(* Logix 5000 Rung export; software revision 16.04 *)

TYPE AFCEModbusGatewayCommand :   // Modbus Gateway Command
STRUCT
   Config : AFCEModbusGatewayConfig;   // Config data to be entered by the user.
   Trigger : BOOL;   // Trigger the Command, when cleared module has responded.
   Data : INT[200];   // Contains modbus data written to the module (write commands)
END_STRUCT
END_TYPE

TYPE AFCEModbusMasterDataType :   // Modbus master data type
STRUCT
   Bit : BOOL;   // bit type
   Word : BOOL;   // word type (16-bit)
   Long : BOOL;   // long integer (32-bit)
   LongRemote : BOOL;   // long integer (32-bit)
END_STRUCT
END_TYPE

TYPE AFCEFlag :   // Flags contains status information updated by ladder and also trigger bits for clock update
STRUCT
   AFCStopped : BOOL;   // Indicates that the module has sent a new input block to be processed by ladder - UPDATED BY LADDER
   AFCInputSequenceNum : INT;   // Meter number (0 -15) associated to blocks 1-16. Used to update "Profile" (meter type and product group.) UPDATED BY LADDER
END_STRUCT
END_TYPE

TYPE AFCEModbusGateway :   // Modbus Gateway
STRUCT
   Command : AFCEModbusGatewayCommand[10];   // Modbus gateway commands - contains setup and modbus data
END_STRUCT
END_TYPE

TYPE AFCEFirmwareVersion :
STRUCT
   Major : SINT;   // Major Version number
   Minor : SINT;   // Minor Version number
   Revision : INT;   // Revision
END_STRUCT
END_TYPE

TYPE AFCEProveConfigEnable :   // Prove controls at enable
STRUCT
   MeterNumber : INT;   // Meter number requested (1-16)
   AutoAcceptProve : BOOL;   // Auto-accept the prove
   AutoContinueProve : BOOL;   // Auto-continue the prove
END_STRUCT
END_TYPE

TYPE AFCEModbusMasterSwap :   // Modbus master swap words/ swap bytes
STRUCT
   SwapWords : BOOL;   // Swap words
   SwapBytes : BOOL;   // Swap bytes
END_STRUCT
END_TYPE

TYPE AFCEUtil :   // Used for internal ladder logic usage. These values must not be changed by user application.
STRUCT
   Flags : AFCEFlag;   // Wallclock update commands
   CycleCounter : INT;   // Reflects current block ID calculated by ladder to be sent to the module
   Buffer : AFCEUtilBuffer;
   Block : AFCEUtilBlock;
END_STRUCT
END_TYPE

TYPE AFCENetworkUTIL :
STRUCT
   State : INT;
   Buffer : SINT[240];
   TimeoutTimer : TIMER;
   TimeoutState : INT;
END_STRUCT
END_TYPE

TYPE AFCEProveConfigAccept :   // Prove controls at accept. If auto-accept is selected must be available at enable
STRUCT
   RequestedInterpolationPoint : INT;   // Requested interpolation point (0 nearest)
   ApplyMFChangeAllStreams : BOOL;   // Apply change in meter factor to all streams
   ApplyMFChangeCurve : BOOL;   // Apply change in meter factor to all curve points
   ApplyNewMF : BOOL;   // CApply new meter factor
END_STRUCT
END_TYPE

TYPE AFCEUtilBlockNonInterrupt :
STRUCT
   Now : BOOL;
   ModbusMasterCommand : BOOL;
   ModbusMasterResponse : BOOL;
   Archive : DINT;
   Prover : BOOL;
   PassThru : BOOL;
   Calibration : BOOL;
END_STRUCT
END_TYPE

TYPE AFCEProve :   // Prove
STRUCT
   Process : AFCEProveProcess;   // Process Variables
   Signals : AFCEProveSignals;   // AFC Prove Signals (triggers the proving update)
   Config : AFCEProveConfig;   // AFC Prove Control (configuration settings)
   PulseCounts : AFCEProvePulseCount;   // Pulse counts to be updated at the end of the run/pass
   ConfigInput : AFCEProveInputConfig;   // AFC prover input configuration
   Status : AFCEProveStatus;   // AFC prover status
   ErrorCode : INT;   // Prove error code
   ProveControlsEcho : INT;   // AFC module Echos the state of the Prove Controls
   RequestedMeterEcho : INT;   // AFC module Echos the Meter number requested
   RequestedCurvePointEcho : INT;   // AFC module Echos the requested Curve Point
   RunResults : AFCEProveRunResults;   // Prove and run results
   ProveEnabled : BOOL;   // ON if prove is enabled. This flag is coped from inputbuffer[247]
END_STRUCT
END_TYPE

TYPE AFCEWallclock :
STRUCT
   GetAFCTime : BOOL;   // Get current AFC Time
   SetAFCTimeFromPLCTime : BOOL;   // Set AFC time from PLC time. Updates current AFC time
   EnableLocalDateTime : BOOL;   // Enable Local Date Time.
   AFCTime : AFCETime;   // Coordinated Universal Time. Updated by either getting or setting AFC time.
END_STRUCT
END_TYPE

TYPE AFCESiteStatus :   // Site status bits - contains general information about the module - not meter specific
STRUCT
   AFCActive : BOOL;   // AFC active
   ChecksumAlarms : BOOL;   // Checkum alarm active
   Reserved2 : BOOL;
   Reserved3 : BOOL;
   PLCHalted : BOOL;   // PLC in program mode or missing
   CfgChanged : BOOL;   // Configuration changed
   Powerup : BOOL;   // Module powered up
   ColdStart : BOOL;   // Module performed cold start (BBRAM initialized)
   ModbusMasterPending : BOOL;   // Modbus Master Poll Pending
   ModbusMasterComplete : BOOL;   // Modbus Master Poll Complete
   ModbusPassThruPending : BOOL;   // Modbus Pass-thru Input Pending
   CalibrationRequest : BOOL;   // Calibration request from module
   ProverEnabled : BOOL;   // Prover Enabled
   Reserved13 : BOOL;
   Reserved14 : BOOL;
   Reserved15 : BOOL;
END_STRUCT
END_TYPE

TYPE AFCEModbusMasterConfig :   // Modbus master command settings
STRUCT
   Enable : BOOL;   // Set to 1 to enable command (0=disable)
   FunctionType : BOOL;   // Set to 1 to select write command (0=read command)
   RegisterBank : BOOL;   // Set to 1 to select input register (0=holding register)
   DataType : AFCEModbusMasterDataType;   // Select data type format
   SwapOption : AFCEModbusMasterSwap;   // Select byte and word swap (1 = swap, 0 = no swap)
   TypeSwap : INT;   // This value is calculated by ladder logic and must not be modified by user
   SlaveAddress : INT;   // Modbus slave address of remote device
   ModbusAddress : INT;   // Modbus data address on remote slave
   ElementCount : INT;   // Number of data elements (125 words)
   TransactionID : INT;   // Transaction ID. This value is returned to the ReturnedTransaction ID when the response has been received.
END_STRUCT
END_TYPE

TYPE AFCEProvePulseCount :   // Values to be supplied at the end of the pass/run
STRUCT
   Meter : DINT;   // Meter pulse count
   MasterMeter : DINT;   // Master meter pulse count
END_STRUCT
END_TYPE

TYPE AFCEUtilBuffer :   // Buffer
STRUCT
   Input : INT[250];   // Input buffer contains the complete block to be copied from the module
   Output : INT[248];   // Output buffer contains data the complete block to be copied to the module
   Process : INT[240];
   ArchiveDay : INT[98];
   ArchiveHour : INT[98];
   Prove : INT[26];
   Analysis : INT[198];
   MeterEnableDisable : INT[4];
   StreamEnable : INT[48];
   StreamDisable : INT[48];
   StreamSelect : INT[32];
   MeterSignals : INT[32];
   Calibration : INT[36];
END_STRUCT
END_TYPE

TYPE AFCEModbusPassThru :   // AFC Modbus Pass-thru
STRUCT
   Enable : BOOL;   // Set to 1 to enable pass-thru functionality (requires AFC Manager setting)
   MessagePresent : BOOL;   // Message present in the response block
   GetMessage : BOOL;   // Get the pass-thru message. When the bit is cleared the message has been transferred to the PLC.
   FunctionBitWrite : BOOL;   // Function bit write
   OverflowError : BOOL;   // Overflow error flag
   ModbusAddress : INT;   // Destination modbus address
   RegisterCount : INT;   // Number of elements associated to command
   ReadDataWord : INT[125];   // Contains received data for word commands
   ReadDataBit : AFCEModbusPassThruBitData;   // Contains received data for bit commands
END_STRUCT
END_TYPE

TYPE AFCEModbusGatewayConfig :   // Modbus Ggateway Configuration
STRUCT
   Enable : BOOL;   // Set to 1 to enable modbus gateway command (0=disable)
   StartRegister : DINT;   // Start modbus address
   RegisterCount : INT;   // Word count (200 max)
   FunctionType : BOOL;   // 0 = read command, 1 = write command
   RegisterType : BOOL;   // 0 = holding register, 1 = input register
   SlaveType : BOOL;   // 0 = primary slave, 1 = virtual slave
END_STRUCT
END_TYPE

TYPE AFCEUtilBlockInterrupt :
STRUCT
   Now : BOOL;
   ModbusGateway : DINT;
   EnableDisable : BOOL;
   Analysis : DINT;
END_STRUCT
END_TYPE

TYPE AFCEModbusMasterCommand :   // Modbus Master Command
STRUCT
   Config : AFCEModbusMasterConfig;   // Modbus Master Configuration
   ErrorCode : INT;   // Error Code associated to Modbus Master Command
   Pending : BOOL;   // Pending Modbus Master Command - waiting for Modbus Response
   ReturnedTransactionID : DINT;   // Changes to Config.TransactionID value when response has returned.
   Data : INT[100];   // Read or Write Data
END_STRUCT
END_TYPE

TYPE AFCEProveStatus :   // Status of the prove (returned from the module to the processor)
STRUCT
   ProveAccepted : BOOL;   // Prove was accepted
   MeterFactorApplied : BOOL;   // Meter factor was applied
   MFAppliedToCurve : BOOL;   // Meter factor was applied to all points in the curve
   MFAppliedToStreams : BOOL;   // Meter factor was applied to all streams
   ProveRejectedByCommand : BOOL;   // Prove was rejected by command
   ProveRejectedNoRuns : BOOL;   // Prove was rejected - empty prove (no runs)
   ProveRejectedDivideBy0 : BOOL;   // Prove was rejected - divide by 0
   ProveEnabled : BOOL;   // Prove is enabled
   ProvingRunInProgress : BOOL;   // Proving run is in progress
   ProveRejectedAbort : BOOL;   // Prove rejected: abort
   ProvePaused : BOOL;   // Prove is paused
   RunCancelled : BOOL;   // Run Is cancelled
   RunTimedOut : BOOL;   // Run timed out
END_STRUCT
END_TYPE

TYPE AFCETime :   // AFC time format used for wallclock update.
STRUCT
   Year : DINT;   // Year
   Month : DINT;   // Month
   Day : DINT;   // Day
   Hour : DINT;   // Hour
   Minute : DINT;   // Minute
   second : DINT;   // Seconds
END_STRUCT
END_TYPE

TYPE AFCEModbusPassThruBitData :   // AFC Modbus Pass-thru Bit Data
STRUCT
   Data : BOOL[2016];   // Contains received data for bit commands
END_STRUCT
END_TYPE

TYPE AFCENetworkConfig :
STRUCT
   GatewayIndex : DINT;
   Physical_Interface_IP : INT[4];
   Physical_Interface_Network_Prefix : SINT;
   Default_Gateway_IP : INT[4];   // The IP address of the gateway. Must be in the same network as the web interface, or null.
   Server1_Network_Prefix : SINT;   // The network prefix length (number of subnet mask bits) of the interface for server 1; a number between 0 and 32.
   Server1_MBAP_Port : DINT;   // The Modbus-TCP port for server 1; 502, or a number between 1024 and 65535.
   Server1_Listener_IP : INT[4];   // The IP address of the network interface for server 1.
END_STRUCT
END_TYPE

TYPE AFCEProveSequencing :   // AFC prove sequencing tag for phase selection and ball positioning
STRUCT
   Phase : AFCEProvePhaseBitmap;   // AFC phase sequencing
   BallPositionReady : BOOL;   // Ball position: Ready (Udir & Bdir only; fwd leg Bdir)
   BallPositionSealed : BOOL;   // Ball position: Sealed (Udir & Bdir only; fwd leg Bdir)
   BallPositionReadyBwdLeg : BOOL;   // Ball position: Ready bwd leg (Bdir only)
   BallPositionSealedBwdLeg : BOOL;   // Ball position: Sealed bwd leg (Bdir only)
END_STRUCT
END_TYPE

TYPE AFCEModbusMaster :   // Modbus Master. Port 3 must be configured as modbus master through AFC Manager to use this feature.
STRUCT
   Enable : BOOL;   // Enable the modbus master funcionality
   CommandIndex : INT;   // Selects which command index will be executed
   Command : AFCEModbusMasterCommand[10];   // Each command contains a specific modbus request to be sent out of the port
END_STRUCT
END_TYPE

TYPE AFCESiteAlarms :   // Indicates if a meter has any alarms
STRUCT
   Meter1 : BOOL;   // Meter in alarm
   Meter2 : BOOL;   // Meter in alarm
   Meter3 : BOOL;   // Meter in alarm
   Meter4 : BOOL;   // Meter in alarm
   Meter5 : BOOL;   // Meter in alarm
   Meter6 : BOOL;   // Meter in alarm
   Meter7 : BOOL;   // Meter in alarm
   Meter8 : BOOL;   // Meter in alarm
   Meter9 : BOOL;   // Meter in alarm
   Meter10 : BOOL;   // Meter in alarm
   Meter11 : BOOL;   // Meter in alarm
   Meter12 : BOOL;   // Meter in alarm
   Meter13 : BOOL;   // Meter in alarm
   Meter14 : BOOL;   // Meter in alarm
   Meter15 : BOOL;   // Meter in alarm
   Meter16 : BOOL;   // Meter in alarm
END_STRUCT
END_TYPE

TYPE AFCEProveSignals :   // Contains the proving signals that will trigger specific tasks from the module
STRUCT
   EnableProve : BOOL;   // Enables the prove
   AcceptProve : BOOL;   // Accepts the prove
   RejectProve : BOOL;   // Reject the prove
   RunStart : BOOL;   // Starts the run
   RunComplete : BOOL;   // Flags that the run is complete
   RunCancel : BOOL;   // Cancels the run
   RunDelete : BOOL;   // Deletes the run
   PassComplete : BOOL;   // Flag that the pass is complete
   PauseProve : BOOL;   // Pauses the Proving Process
   AbortProve : BOOL;   // Aborts the prove
END_STRUCT
END_TYPE

TYPE AFCEProvePhaseBitmap :   // AFC prove phase bitmap
STRUCT
   NotSelected : BOOL;   // Not selected
   Active : BOOL;   // Active, not counting
   CountingPast1stSwitch : BOOL;   // Counting past 1st switch for Udir and forward leg for Bdir)
   Past2ndSwitchFwdLeg : BOOL;   // Past 2nd switch forward leg (bidirectional only)
   Past1stSwithRetLeg : BOOL;   // Past 1st switch return leg (bidirectional only)
   RunComplete : BOOL;   // Run complete. past 2nd switch.
END_STRUCT
END_TYPE

TYPE AFCEUtilBlock :
STRUCT
   ProcessInput : INT;
   InterruptPending : AFCEUtilBlockInterrupt;
   InterruptComplete : AFCEUtilBlockInterrupt;
   NonInterruptPending : AFCEUtilBlockNonInterrupt;
   NonInterruptComplete : AFCEUtilBlockNonInterrupt;
END_STRUCT
END_TYPE

TYPE AFCEProveProcess :   // Prove process output from processor to the module
STRUCT
   Sequencing : AFCEProveSequencing;   // Prover sequencing
   Temperature : REAL;   // Temperature for Single Probe provers. And Inlet Temperature for Dual Probe Provers.
   OutletTemperature : REAL;   // Outlet Temperature for Provers with Dual Probes.
   SwitchBarTemperature : REAL;   // Switch bar temperature
   Pressure : REAL;   // Pressure for Single Probe provers. And Inlet Pressure for Dual Probe Provers.
   OutletPressure : REAL;   // Outlet Pressure for Provers with Dual Probes.
   ProverDensity : REAL;   // Prover density
END_STRUCT
END_TYPE

TYPE AFCENetwork :
STRUCT
   Read : BOOL;   // Trigger to read network parameters
   Write : BOOL;   // Trigger to write network parameters
   Config : AFCENetworkConfig;   // Network parameters
   Error : INT;   // 0 = OK, -1 = Timeout, -2 = Gateway Index Out of Range
   Util : AFCENetworkUTIL;   // Internal variables
END_STRUCT
END_TYPE

TYPE AFCEProveInputConfig :   // Prove input block results - prover configuration
STRUCT
   Type : INT;   // Prover type
   Options : INT;   // Prover options
   RunsPerProveTotal : INT;   // Total runs per prove
   RunsPerProveSelected : INT;   // Selected runs per prove
   MaxRunsBeforeAbort : INT;   // Max total runs before abort
   ShortPassesPerRun : INT;   // Short passes per run if bidir = 2 , else 0
END_STRUCT
END_TYPE

TYPE AFCEProveConfig :   // Controls (configuration settings) associated to the prover
STRUCT
   Enable : AFCEProveConfigEnable;   // Controls at enable
   Accept : AFCEProveConfigAccept;   // Controls at accept
END_STRUCT
END_TYPE

TYPE AFCEModuleDef :   // Main user defined data type
STRUCT
   ModbusGateway : AFCEModbusGateway;   // Reads and write data between processor and module modbus table
   ModbusMaster : AFCEModbusMaster;   // Setup modbus master commands to be sent to remote slaves (through Port 3)
   ModbusPassThru : AFCEModbusPassThru;   // Modbus pass-thru data
   SiteStatus : AFCESiteStatus;   // Site status
   MeterAlarms : AFCESiteAlarms;   // Meter Alarms
   Prove : AFCEProve;   // Prover
   Wallclock : AFCEWallclock;   // Set clock and get clock information
   Firmware : AFCEFirmwareVersion;   // Firmware information
   Util : AFCEUtil;   // Used by ladder logic
END_STRUCT
END_TYPE

TYPE AFCEProveRunResults :   // Run results of the prove. Copied from the module to the pocessor
STRUCT
   CountAttempted : INT;   // Run count attempted
   CountCompleted : INT;   // Run count completed
   CountSelected : INT;   // Run count selected
   RunsSelected : INT;   // Bit Mapped Runs selected for calculations from completed runs
   NewMeterFactor : REAL;   // New meter factor
   ChangeInMeterFactor : REAL;   // Change in meter factor
END_STRUCT
END_TYPE

ADD_ON_INSTRUCTION AOI56EAFCNetworkConfig   (* revision 1.1, ExecutePrescan *)
// Add-On instruction to update the MVI56E-AFC network settings
// Revision note:
// Made changes to the ModbusGatewayConfig UDT StartRegister Tag Data Type from INT to DINT.
// Help:
// v1.0: Read and write module network configuration.
// v1.1: Made changes to the ModbusGatewayConfig UDT StartRegister Tag Data Type from INT to DINT.
VAR_IN_OUT
   Network : AFCENetwork; {required}
   EAFC : AFCEModuleDef; {required}
END_VAR
VAR
   NetworkBuffer : DINT[2];
   MVMbuffer : INT;
   IndexSizeM1 : DINT;
   IndexSize : DINT;
   Index : DINT;
   ErrorTimer : TIMER;
END_VAR

ROUTINE Logic   (* ladder *)
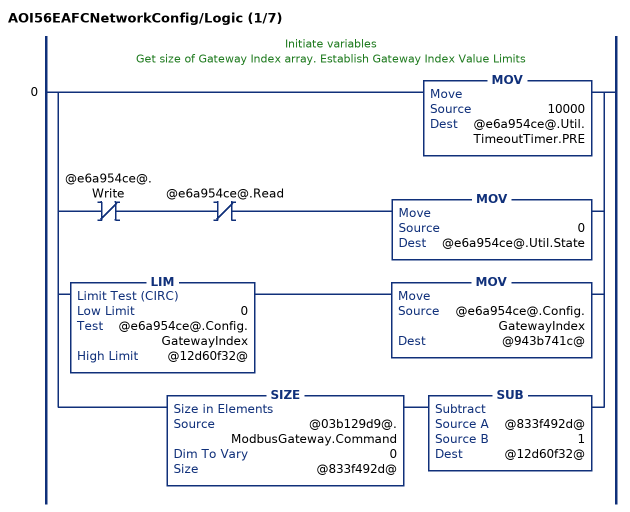
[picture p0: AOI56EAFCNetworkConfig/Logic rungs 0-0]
   // Initiate variables
   // Get size of Gateway Index array. Establish Gateway Index Value Limits
   0: [[MOV(10000,@e6a954ce@.Util.TimeoutTimer.PRE) ,XIO(@e6a954ce@.Write) XIO(@e6a954ce@.Read) MOV(0,@e6a954ce@.Util.State) ] ,LIM(0,@e6a954ce@.Config.GatewayIndex,@12d60f32@) MOV(@e6a954ce@.Config.GatewayIndex,@943b741c@) ,SIZE(@03b129d9@.ModbusGateway.Command,0,@833f492d@) SUB(@833f492d@,1,@12d60f32@) ];
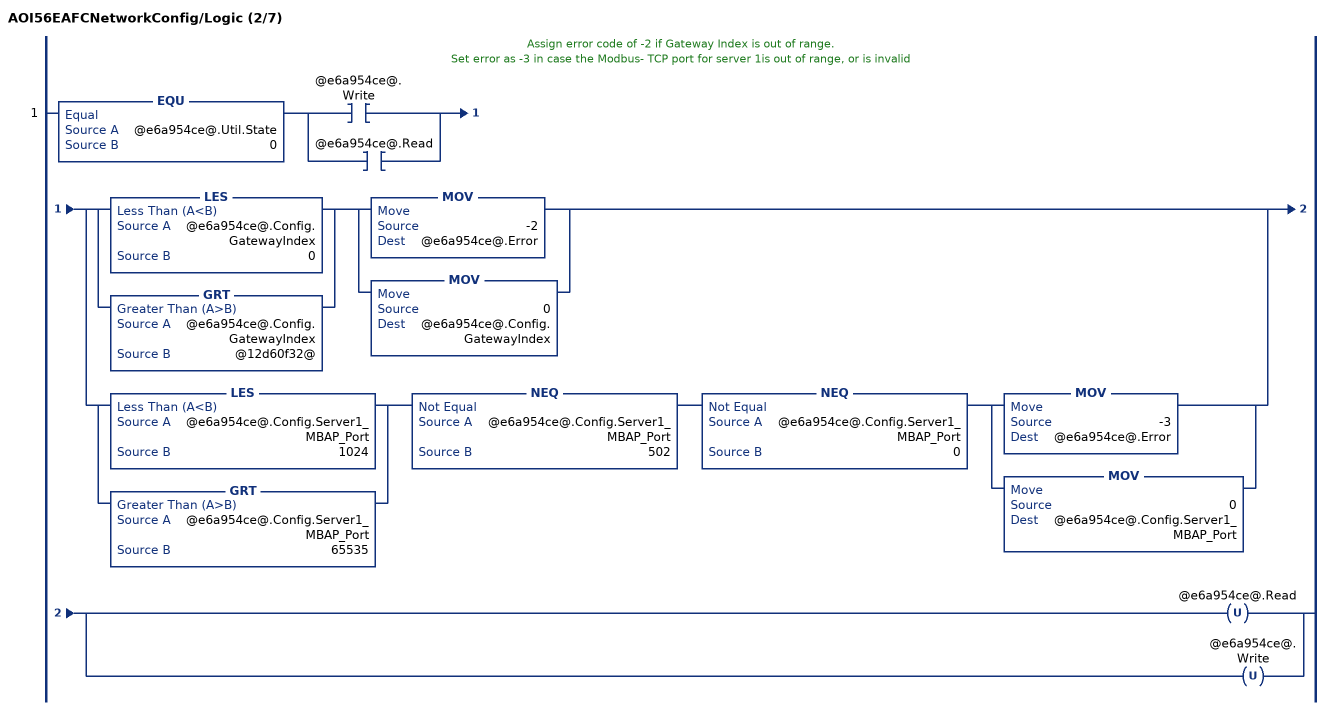
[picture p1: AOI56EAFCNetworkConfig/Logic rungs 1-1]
   // Assign error code of -2 if Gateway Index is out of range.
   // Set error as -3 in case the Modbus- TCP port for server 1is out of range, or is invalid
   1: EQU(@e6a954ce@.Util.State,0)[XIC(@e6a954ce@.Write) ,XIC(@e6a954ce@.Read) ][[LES(@e6a954ce@.Config.GatewayIndex,0) ,GRT(@e6a954ce@.Config.GatewayIndex,@12d60f32@) ] [MOV(-2,@e6a954ce@.Error) ,MOV(0,@e6a954ce@.Config.GatewayIndex) ] ,[LES(@e6a954ce@.Config.Server1_MBAP_Port,1024) ,GRT(@e6a954ce@.Config.Server1_MBAP_Port,65535) ] NEQ(@e6a954ce@.Config.Server1_MBAP_Port,502) NEQ(@e6a954ce@.Config.Server1_MBAP_Port,0) [MOV(-3,@e6a954ce@.Error) ,MOV(0,@e6a954ce@.Config.Server1_MBAP_Port) ] ][OTU(@e6a954ce@.Read) ,OTU(@e6a954ce@.Write) ];
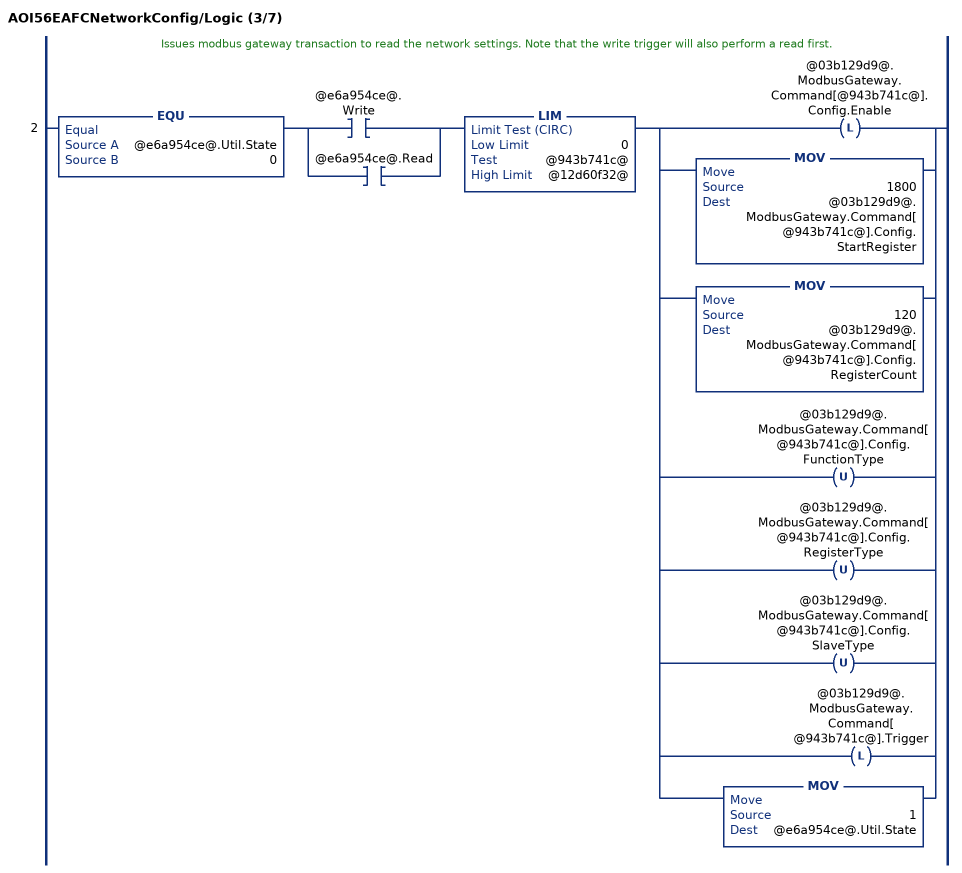
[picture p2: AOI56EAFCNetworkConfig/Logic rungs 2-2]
   // Issues modbus gateway transaction to read the network settings. Note that the write trigger will also perform a read first.
   2: EQU(@e6a954ce@.Util.State,0)[XIC(@e6a954ce@.Write) ,XIC(@e6a954ce@.Read) ]LIM(0,@943b741c@,@12d60f32@)[OTL(@03b129d9@.ModbusGateway.Command[@943b741c@].Config.Enable) ,MOV(1800,@03b129d9@.ModbusGateway.Command[@943b741c@].Config.StartRegister) ,MOV(120,@03b129d9@.ModbusGateway.Command[@943b741c@].Config.RegisterCount) ,OTU(@03b129d9@.ModbusGateway.Command[@943b741c@].Config.FunctionType) ,OTU(@03b129d9@.ModbusGateway.Command[@943b741c@].Config.RegisterType) ,OTU(@03b129d9@.ModbusGateway.Command[@943b741c@].Config.SlaveType) ,OTL(@03b129d9@.ModbusGateway.Command[@943b741c@].Trigger) ,MOV(1,@e6a954ce@.Util.State) ];
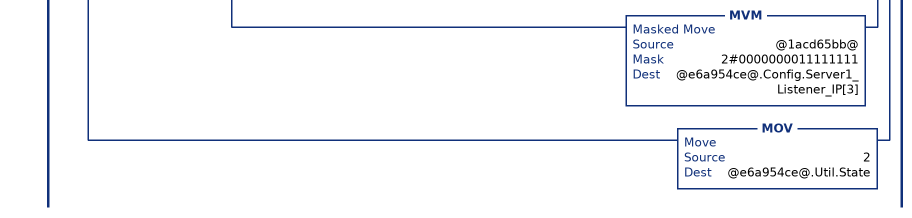
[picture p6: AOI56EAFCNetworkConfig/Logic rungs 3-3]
   // Parses the data received from the module once it detects that the gateway transaction was concluded.
   3: EQU(@e6a954ce@.Util.State,1)[XIC(@e6a954ce@.Write) ,XIC(@e6a954ce@.Read) ]XIO(@03b129d9@.ModbusGateway.Command[@943b741c@].Trigger)LIM(0,@943b741c@,@12d60f32@)[COP(@03b129d9@.ModbusGateway.Command[@943b741c@].Data[0],@e6a954ce@.Util.Buffer[0],240) ,XIC(@e6a954ce@.Read) [COP(@e6a954ce@.Util.Buffer[3],@1acd65bb@,1) ,MVM(@1acd65bb@,2#0000000011111111,@e6a954ce@.Config.Physical_Interface_IP[0]) ,COP(@e6a954ce@.Util.Buffer[2],@1acd65bb@,1) ,MVM(@1acd65bb@,2#0000000011111111,@e6a954ce@.Config.Physical_Interface_IP[1]) ,COP(@e6a954ce@.Util.Buffer[1],@1acd65bb@,1) ,MVM(@1acd65bb@,2#0000000011111111,@e6a954ce@.Config.Physical_Interface_IP[2]) ,COP(@e6a954ce@.Util.Buffer[0],@1acd65bb@,1) ,MVM(@1acd65bb@,2#0000000011111111,@e6a954ce@.Config.Physical_Interface_IP[3]) ,MOV(@e6a954ce@.Util.Buffer[4],@e6a954ce@.Config.Physical_Interface_Network_Prefix) ,COP(@e6a954ce@.Util.Buffer[15],@1acd65bb@,1) ,MVM(@1acd65bb@,2#0000000011111111,@e6a954ce@.Config.Default_Gateway_IP[0]) ,COP(@e6a954ce@.Util.Buffer[14],@1acd65bb@,1) ,MVM(@1acd65bb@,2#0000000011111111,@e6a954ce@.Config.Default_Gateway_IP[1]) ,COP(@e6a954ce@.Util.Buffer[13],@1acd65bb@,1) ,MVM(@1acd65bb@,2#0000000011111111,@e6a954ce@.Config.Default_Gateway_IP[2]) ,COP(@e6a954ce@.Util.Buffer[12],@1acd65bb@,1) ,MVM(@1acd65bb@,2#0000000011111111,@e6a954ce@.Config.Default_Gateway_IP[3]) ,MOV(@e6a954ce@.Util.Buffer[20],@e6a954ce@.Config.Server1_Network_Prefix) ,COP(@e6a954ce@.Util.Buffer[26],@c24fad98@[0],2) MVM(@c24fad98@[0],2#00000000000000001111111111111111,@e6a954ce@.Config.Server1_MBAP_Port) ,COP(@e6a954ce@.Util.Buffer[31],@1acd65bb@,1) ,MVM(@1acd65bb@,2#0000000011111111,@e6a954ce@.Config.Server1_Listener_IP[0]) ,COP(@e6a954ce@.Util.Buffer[30],@1acd65bb@,1) ,MVM(@1acd65bb@,2#0000000011111111,@e6a954ce@.Config.Server1_Listener_IP[1]) ,COP(@e6a954ce@.Util.Buffer[29],@1acd65bb@,1) ,MVM(@1acd65bb@,2#0000000011111111,@e6a954ce@.Config.Server1_Listener_IP[2]) ,COP(@e6a954ce@.Util.Buffer[28],@1acd65bb@,1) ,MOV(0,@e6a954ce@.Error) ,MVM(@1acd65bb@,2#0000000011111111,@e6a954ce@.Config.Server1_Listener_IP[3]) ] ,MOV(2,@e6a954ce@.Util.State) ];
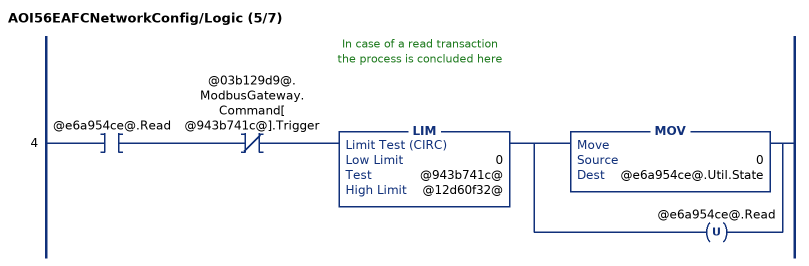
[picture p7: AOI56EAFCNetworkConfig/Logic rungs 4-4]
   // In case of a read transaction
   //  the process is concluded here
   4: XIC(@e6a954ce@.Read)XIO(@03b129d9@.ModbusGateway.Command[@943b741c@].Trigger)LIM(0,@943b741c@,@12d60f32@)[MOV(0,@e6a954ce@.Util.State) ,OTU(@e6a954ce@.Read) ];
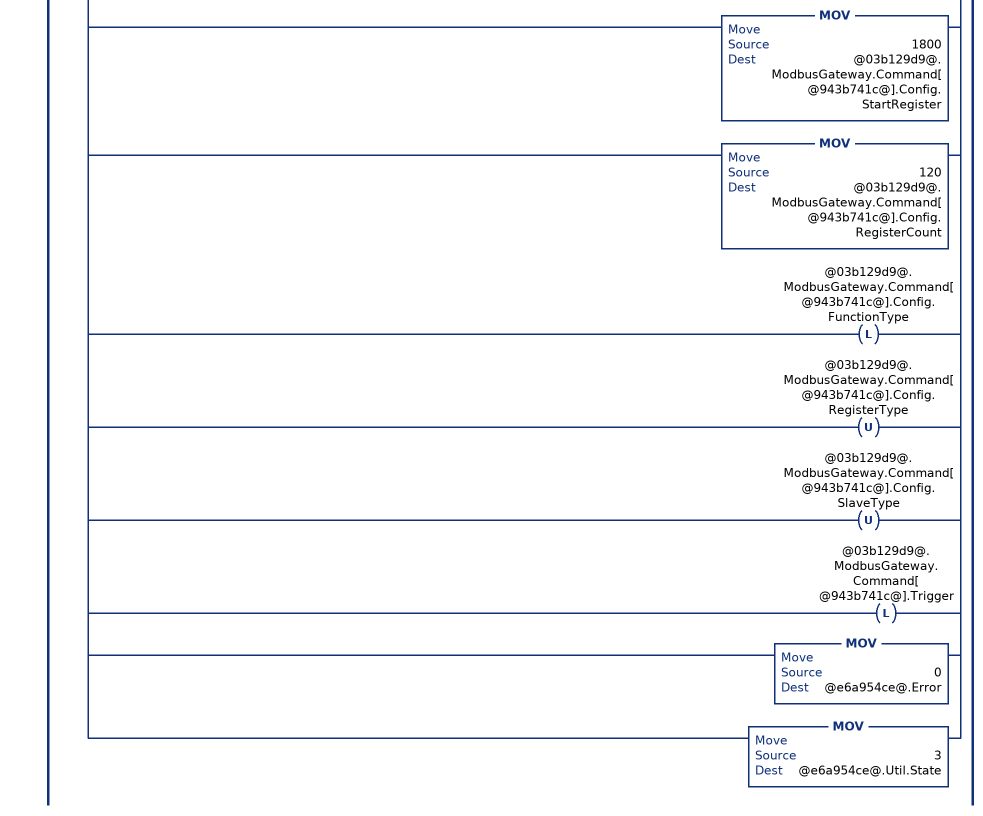
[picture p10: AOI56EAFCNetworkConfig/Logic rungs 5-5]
   // In case this is a write transaction
   //  this rung will update the the specific parameters listed at Network.Config and keep the remaining data the same as read from the module.
   5: EQU(@e6a954ce@.Util.State,2)[LIM(1024,@e6a954ce@.Config.Server1_MBAP_Port,65535) ,EQU(@e6a954ce@.Config.Server1_MBAP_Port,502) ]LIM(0,@943b741c@,@12d60f32@)XIC(@e6a954ce@.Write)[COP(@e6a954ce@.Config.Physical_Interface_IP[0],@e6a954ce@.Util.Buffer[3],1) ,COP(@e6a954ce@.Config.Physical_Interface_IP[1],@e6a954ce@.Util.Buffer[2],1) ,COP(@e6a954ce@.Config.Physical_Interface_IP[2],@e6a954ce@.Util.Buffer[1],1) ,COP(@e6a954ce@.Config.Physical_Interface_IP[3],@e6a954ce@.Util.Buffer[0],1) ,MOV(@e6a954ce@.Config.Physical_Interface_Network_Prefix,@e6a954ce@.Util.Buffer[4]) ,COP(@e6a954ce@.Config.Default_Gateway_IP[0],@e6a954ce@.Util.Buffer[15],1) ,COP(@e6a954ce@.Config.Default_Gateway_IP[1],@e6a954ce@.Util.Buffer[14],1) ,COP(@e6a954ce@.Config.Default_Gateway_IP[2],@e6a954ce@.Util.Buffer[13],1) ,COP(@e6a954ce@.Config.Default_Gateway_IP[3],@e6a954ce@.Util.Buffer[12],1) ,MOV(@e6a954ce@.Config.Server1_Network_Prefix,@e6a954ce@.Util.Buffer[20]) ,COP(@e6a954ce@.Config.Server1_MBAP_Port,@e6a954ce@.Util.Buffer[26],2) ,COP(@e6a954ce@.Config.Server1_Listener_IP[0],@e6a954ce@.Util.Buffer[31],1) ,COP(@e6a954ce@.Config.Server1_Listener_IP[1],@e6a954ce@.Util.Buffer[30],1) ,COP(@e6a954ce@.Config.Server1_Listener_IP[2],@e6a954ce@.Util.Buffer[29],1) ,COP(@e6a954ce@.Config.Server1_Listener_IP[3],@e6a954ce@.Util.Buffer[28],1) ,COP(@e6a954ce@.Util.Buffer[0],@03b129d9@.ModbusGateway.Command[@943b741c@].Data[0],120) ,MOV(1800,@03b129d9@.ModbusGateway.Command[@943b741c@].Config.StartRegister) ,MOV(120,@03b129d9@.ModbusGateway.Command[@943b741c@].Config.RegisterCount) ,OTL(@03b129d9@.ModbusGateway.Command[@943b741c@].Config.FunctionType) ,OTU(@03b129d9@.ModbusGateway.Command[@943b741c@].Config.RegisterType) ,OTU(@03b129d9@.ModbusGateway.Command[@943b741c@].Config.SlaveType) ,OTL(@03b129d9@.ModbusGateway.Command[@943b741c@].Trigger) ,MOV(0,@e6a954ce@.Error) ,MOV(3,@e6a954ce@.Util.State) ];
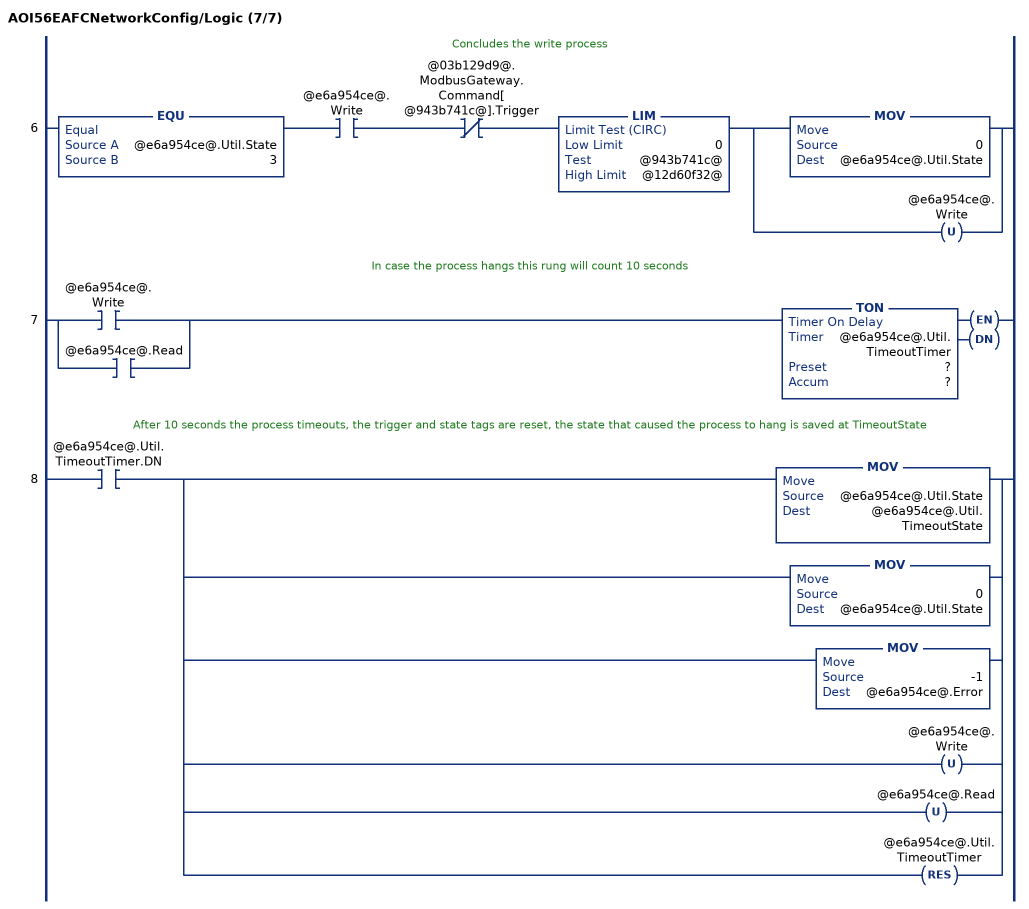
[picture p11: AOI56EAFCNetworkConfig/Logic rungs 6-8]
   // Concludes the write process
   6: EQU(@e6a954ce@.Util.State,3)XIC(@e6a954ce@.Write)XIO(@03b129d9@.ModbusGateway.Command[@943b741c@].Trigger)LIM(0,@943b741c@,@12d60f32@)[MOV(0,@e6a954ce@.Util.State) ,OTU(@e6a954ce@.Write) ];
   // In case the process hangs this rung will count 10 seconds
   7: [XIC(@e6a954ce@.Write) ,XIC(@e6a954ce@.Read) ]TON(@e6a954ce@.Util.TimeoutTimer,?,?);
   // After 10 seconds the process timeouts, the trigger and state tags are reset, the state that caused the process to hang is saved at TimeoutState
   8: XIC(@e6a954ce@.Util.TimeoutTimer.DN)[MOV(@e6a954ce@.Util.State,@e6a954ce@.Util.TimeoutState) ,MOV(0,@e6a954ce@.Util.State) ,MOV(-1,@e6a954ce@.Error) ,OTU(@e6a954ce@.Write) ,OTU(@e6a954ce@.Read) ,RES(@e6a954ce@.Util.TimeoutTimer) ];
END_ROUTINE

ROUTINE Prescan   (* ladder *)
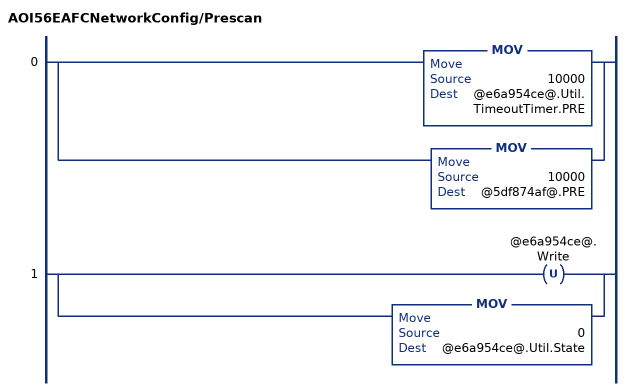
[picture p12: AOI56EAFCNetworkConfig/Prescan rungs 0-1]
   0: [MOV(10000,@e6a954ce@.Util.TimeoutTimer.PRE) ,MOV(10000,@5df874af@.PRE) ];
   1: [OTU(@e6a954ce@.Write) ,MOV(0,@e6a954ce@.Util.State) ];
END_ROUTINE
END_ADD_ON_INSTRUCTION

VAR_GLOBAL   (* controller tags *)
   Network : AFCENetwork;
   AFC : AFCEModuleDef;
   AOINetworkConfig : AOI56EAFCNetworkConfig;
END_VAR

PROGRAM MainProgram

ROUTINE MainRoutine   (* ladder *)
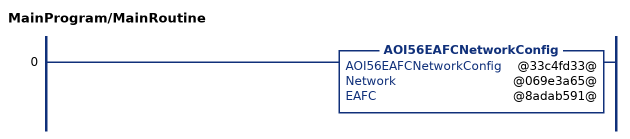
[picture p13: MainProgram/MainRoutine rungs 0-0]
   0: AOI56EAFCNetworkConfig(@33c4fd33@,@069e3a65@,@8adab591@);
END_ROUTINE
END_PROGRAM
